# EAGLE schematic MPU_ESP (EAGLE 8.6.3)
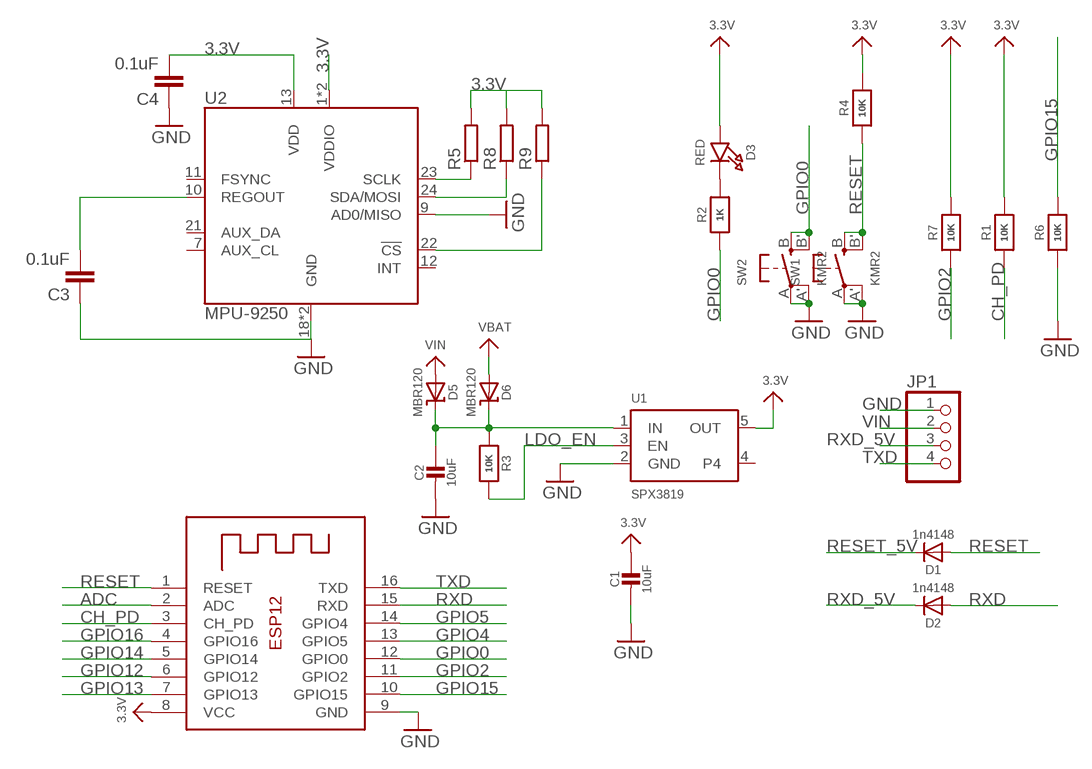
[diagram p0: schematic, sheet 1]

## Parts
C1  10uF  CAP_CERAMIC0805-NOOUTLINE  [0805-NO]
C2  10uF  CAP_CERAMIC0805-NOOUTLINE  [0805-NO]
C3  0.1uF  C  [C0805]
C4  0.1uF  C  [C0805]
D1  1n4148  DIODESOD-323  [SOD-323]
D2  1n4148  DIODESOD-323  [SOD-323]
D3  RED  LED0805_NOOUTLINE  [CHIPLED_0805_NOOUTLINE]
D5  MBR120  DIODE-SCHOTTKYSOD-123  [SOD-123]
D6  MBR120  DIODE-SCHOTTKYSOD-123  [SOD-123]
JP1  PINHD-1X4/90  [1X04/90]
R1  10K  RESISTOR0805_NOOUTLINE  [0805-NO]
R2  1K  RESISTOR0805_NOOUTLINE  [0805-NO]
R3  10K  RESISTOR0805_NOOUTLINE  [0805-NO]
R4  10K  RESISTOR0805_NOOUTLINE  [0805-NO]
R5  R  [R0805]
R6  10K  RESISTOR0805_NOOUTLINE  [0805-NO]
R7  10K  RESISTOR0805_NOOUTLINE  [0805-NO]
R8  R  [R0805]
R9  R  [R0805]
SW1  KMR2  SWITCH_TACT_SMT4.6X2.8  [BTN_KMR2_4.6X2.8]
SW2  KMR2  SWITCH_TACT_SMT4.6X2.8  [BTN_KMR2_4.6X2.8]
U1  SPX3819  VREG_SOT23-5  [SOT23-5]
U2  MPU-9250  [QFN-24/3MM]
X1  ESP-12  [ESP-12]

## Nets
3.3V: C1.1 C4.2 D3.A R1.2 R4.2 R5.2 R7.2 R8.2 R9.2 U1.5(OUT) U2.1(VDDIO) U2.8(VDDIO) U2.13(VDD) X1.8(VCC)
ADC: X1.2(ADC)
CH_PD: R1.1 X1.3(CH_PD)
GND: C1.2 C2.2 C3.1 C4.1 JP1.1 R6.1 SW1.A'(P1) SW1.A(P) SW2.A'(P1) SW2.A(P) U1.2(GND) U2.9(AD0/MISO) U2.18(GND) U2.20(GND) X1.9(GND)
GPIO0: R2.1 SW2.B'(S1) SW2.B(S) X1.12(GPIO0)
GPIO2: R7.1 X1.11(GPIO2)
GPIO4: X1.13(GPIO5)
GPIO5: X1.14(GPIO4)
GPIO12: X1.6(GPIO12)
GPIO13: X1.7(GPIO13)
GPIO14: X1.5(GPIO14)
GPIO15: R6.2 X1.10(GPIO15)
GPIO16: X1.4(GPIO16)
LDO_EN: R3.2 U1.3(EN)
N$1: D3.C R2.2
N$2: C2.1 D5.C D6.C R3.1 U1.1(IN)
N$3: R9.1 U2.22(!CS)
N$4: R8.1 U2.24(SDA/MOSI)
N$5: R5.1 U2.23(SCLK)
REGOUT: C3.2 U2.10(REGOUT)
RESET: D1.A R4.1 SW1.B'(S1) SW1.B(S) X1.1(RESET)
RESET_5V: D1.C
RXD: D2.A X1.15(RXD)
RXD_5V: D2.C JP1.3
TXD: JP1.4 X1.16(TXD)
VBAT: D6.A
VIN: D5.A JP1.2
Unconnected: U1.4 U2.7(AUX_CL) U2.11(FSYNC) U2.12(INT) U2.21(AUX_DA)

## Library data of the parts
C1 C2 = microbuilder:CAP_CERAMIC: Ceramic Capacitors
C3 C4 = eagle-ltspice:C: CAPACITOR, European symbol; SPICEMODEL: NONE; SPICEPREFIX: C
D1 D2 = microbuilder:DIODE: Diode
D3 = microbuilder:LED: LED
D5 D6 = microbuilder:DIODE-SCHOTTKY
JP1 = pinhead:PINHD-1X4: PIN HEADER
R1-R4 R6 R7 = microbuilder:RESISTOR: Resistors
R5 R8 R9 = eagle-ltspice:R: RESISTOR, European symbol; SPICEMODEL: NONE; SPICEPREFIX: R
SW1 SW2 = microbuilder:SWITCH_TACT_SMT: SMT Tact Switches 6x6mm - Digikey: P12940SCT-ND KMR2 (4.6x2.8mm) - Digikey: 401-1426-1-ND EVQ-PQHB55 - Light Touch, 160GF (4.5x4.5mm) - Digikey: P8090SCT-ND KMT0 - KMT021 NGJ LHS (etc.) IP68/Waterproof - Digikey: CKN10289CT-ND
U1 = microbuilder:VREG_SOT23-5: SOT23-5 Fixed Voltage Regulators Part Current Out V Out V In V Dropout θJA (°C/W) TJ (°C) Digikey Part No. ADP121 150mA 3.3V 3.4-5.5V 0.09V @ 150mA -- -- ADP121-AUJZ33R7CT-ND ADP121 150mA 3.0V 3.1-5.5V 0.09V @ 150mA -- -- ADP121-AUJZ30R7CT-ND ADP122 300mA 3.3V 3.4-5.5V 0.085V @ 300mA -- --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
U2 = MPU-9250:MPU-9250: GYRO/ACCEL/COMPASS/9-AXIS; AVAILABILITY: Good; DESCRIPTION: IMU ACCEL/GYRO/MAG I2C/SPI 24QFN; MF: TDK; MP: MPU-9250; PACKAGE: QFN-24 InvenSense; PRICE: 6.36 USD
X1 = microbuilder:ESP-12

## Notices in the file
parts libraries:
microbuilder: This work is placed in the public domain, and may be freely used for commercial and non-commercial work with the following conditions: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
